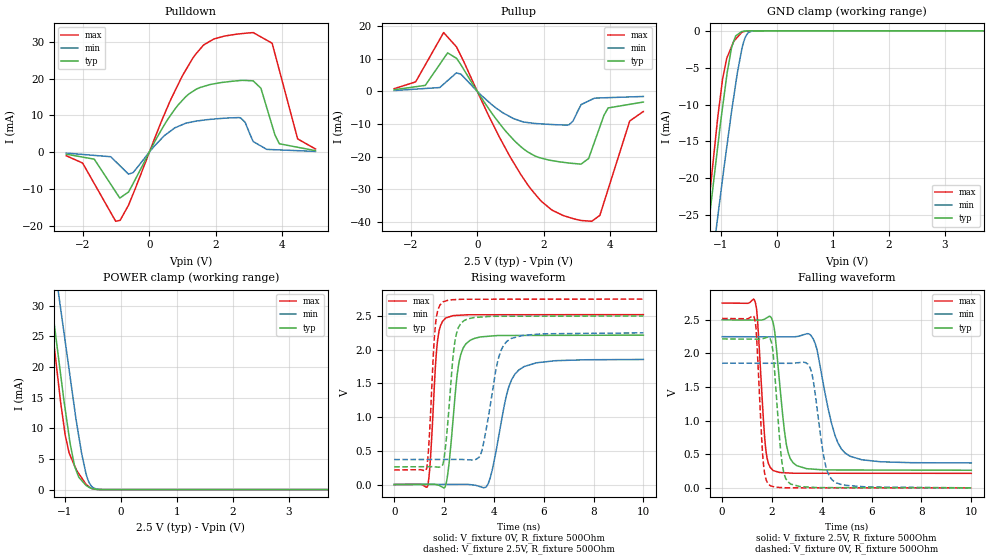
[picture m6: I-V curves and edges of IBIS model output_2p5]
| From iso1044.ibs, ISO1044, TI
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|   output_2p5 Model
[Model]   output_2p5
Model_type   3-state
Polarity   Inverting
Vmeas = 1.25
Vref = 0
Cref = 2pF
Rref = 100000
|   typ   min   max
C_comp   1.246pF   1.207pF   1.335pF
|C_comp_pullup   1.19pF   1.212pF   1.212pF
|C_comp_pulldown   1.131pF   1.152pF   1.158pF
|  Where Nom  PVT is Nominal Process, 2.5V,   27C
|   Fast PVT is Strong Process,  2.75,  -40C
|   Slow PVT is Weak Process,   2.25V,  150C
[Voltage Range]   2.5   2.25   2.75
|Junction Temperature
[Temperature Range]   27   150   -40
[Pullup Reference]   2.5   2.25   2.75
[Pulldown Reference]   -0   -0   0
[Power Clamp Reference]   2.5   2.25   2.75
[GND Clamp Reference]   0   0   0
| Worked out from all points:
|   slope of the pulldown table from 0 to 0.375 V, typ, clamps not added: 60.3 ohm
|   slope of the pullup table from 0 to 0.375 V, typ, clamps not added: 65.2 ohm
|   GND clamp passes 1 mA (typ) near -0.75 V on its own axis
|   POWER clamp passes 1 mA (typ) near -0.65 V on its own axis
|   falling waveform, V_fixture 2.5V, R_fixture 500Ohm: 20-80 % time 368ps typ, 664ps min, 250ps max; typ from 2.5 V to 0.262 V
|   rising waveform, V_fixture 0V, R_fixture 500Ohm: 20-80 % time 347ps typ, 615ps min, 233ps max; typ from 0 V to 2.22 V
|   rising waveform, V_fixture 2.5V, R_fixture 500Ohm: 20-80 % time 310ps typ, 531ps min, 212ps max; typ from 0.262 V to 2.5 V
|   falling waveform, V_fixture 0V, R_fixture 500Ohm: 20-80 % time 283ps typ, 428ps min, 209ps max; typ from 2.22 V to 0 V
[Pulldown]
|   Voltage   I(typ)   I(min)   I(max)
-2.5V     -577uA     -287.9uA   -1.006mA
-1.657V   -1.93mA    -903.9uA   -8.578mA
-879.3mV  -12.45mA   -3.763mA   -18.56mA
-486.8mV  -8.536mA   -5.561mA   -11.35mA
553.4mV   8.878mA    5.156mA    12.39mA
1.381V    16.92mA    8.373mA    26.47mA
2.746V    19.46mA    9.303mA    32.17mA
3.125V    19.37mA    2.86mA     32.5mA
3.696V    7.22mA     667.1uA    29.61mA
3.912V    2.258mA    586.3uA    22.27mA
4.464V    1.309mA    380.2uA    3.573mA
5V        388uA      180.2uA    845.5uA
[GND Clamp]
|   Voltage   I(typ)   I(min)   I(max)
-2.5V     -115.3mA   -116.6mA   -126.4mA
-1.497V   -45.2mA    -52.65mA   -45.36mA
-1.225V   -26.73mA   -35.65mA   -24.1mA
-1.057V   -15.78mA   -25.31mA   -11.83mA
-968.7mV  -10.36mA   -20.06mA   -6.529mA
-896.2mV  -6.193mA   -15.89mA   -3.763mA
-806.5mV  -2.199mA   -10.84mA   -2.1mA
-734.8mV  -686.4uA   -7.22mA    -1.127mA
-625mV    -98.47uA   -2.474mA   -201uA
-538.5mV  -20.04uA   -530.7uA   -38.58uA
-416.7mV  -957.2nA   -25.09uA   -1.059uA
5V        0A         0A         0A
[Pullup]
|   Voltage   I(typ)   I(min)   I(max)
-2.5V     504.9uA    255.7uA    828.2uA
-1.855V   1.423mA    688.6uA    2.91mA
-1.013V   10.01mA    2.217mA    18.02mA
-489.1mV  8.086mA    5.245mA    10.84mA
1.515V    -18.52mA   -9.543mA   -28.54mA
2.76V     -21.95mA   -10.26mA   -38.59mA
3.125V    -22.29mA   -4.049mA   -39.56mA
3.352V    -20.57mA   -2.944mA   -39.73mA
3.69V     -10.88mA   -2.009mA   -38mA
3.939V    -5.079mA   -1.924mA   -30mA
4.589V    -3.972mA   -1.703mA   -9.094mA
5V        -3.272mA   -1.563mA   -6.145mA
[POWER Clamp]
|   Voltage   I(typ)   I(min)   I(max)
-2.5V     128.9mA    131.9mA    138mA
-1.51V    51.07mA    59.94mA    50.15mA
-1.243V   30.77mA    41.03mA    27.33mA
-1.116V   21.48mA    31.98mA    17.2mA
-995.9mV  13.05mA    24.1mA     8.839mA
-926.6mV  8.645mA    19.55mA    5.963mA
-830.5mV  3.863mA    13.25mA    3.946mA
-703.7mV  1.504mA    5.938mA    1.939mA
-571.6mV  367.3uA    1.204mA    444.5uA
-470.7mV  96.86uA    197.6uA    59.09uA
-303.6mV  856.2nA    6.608uA    5.542uA
5V        0A         0A         0A
[Ramp]
R_load = 500
|   typ   min   max
dV/dt_r   1.32944/3.44254e-10   1.11276/6.08998e-10   1.51209/2.31266e-10
dV/dt_f   1.34275/3.66094e-10   1.12742/6.60572e-10   1.52035/2.48834e-10
[Falling Waveform]
V_fixture = 2.5V
V_fixture_min = 2.25V
V_fixture_max = 2.75V
R_fixture = 500Ohm
C_fixture = 0F
|   Time   V(typ)   V(min)   V(max)
0s        2.5V       2.25V      2.75V
1.327ns   2.497V     2.248V     2.768V
1.745ns   2.52V      2.248V     599.3mV
2.045ns   2.46V      2.247V     260.3mV
2.571ns   664.8mV    2.247V     223.3mV
2.981ns   333.5mV    2.251V     217.8mV
3.733ns   276.2mV    2.15V      217.6mV
4.389ns   266.3mV    962.5mV    217.4mV
4.929ns   265.9mV    520.9mV    217.3mV
10ns      262.1mV    370.6mV    216.1mV
[Rising Waveform]
V_fixture = 0V
V_fixture_min = 0V
V_fixture_max = 0V
R_fixture = 500Ohm
C_fixture = 0F
|   Time   V(typ)   V(min)   V(max)
0s        -149.7nV   307.1uV    -128.4nV
1.341ns   2.6mV      1.279mV    -24.13mV
1.725ns   -5.249mV   1.557mV    2.084V
2.065ns   -10.42mV   1.803mV    2.468V
2.591ns   1.792V     2.184mV    2.51V
3.041ns   2.137V     -1.144mV   2.518V
3.78ns    2.199V     19.03mV    2.518V
4.509ns   2.211V     1.329V     2.518V
4.999ns   2.211V     1.699V     2.519V
10ns      2.216V     1.855V     2.52V
[Rising Waveform]
V_fixture = 2.5V
V_fixture_min = 2.25V
V_fixture_max = 2.75V
R_fixture = 500Ohm
C_fixture = 0F
|   Time   V(typ)   V(min)   V(max)
0s        262.1mV    370.6mV    216.1mV
1.298ns   264.3mV    371.2mV    232.3mV
1.647ns   261.8mV    371.4mV    2.339V
1.945ns   293mV      371.5mV    2.706V
2.431ns   2.108V     371.7mV    2.743V
2.801ns   2.431V     370.2mV    2.748V
3.463ns   2.484V     439.7mV    2.749V
4.13ns    2.496V     1.789V     2.749V
4.519ns   2.496V     2.123V     2.749V
10ns      2.5V       2.25V      2.75V
[Falling Waveform]
|Gnd
V_fixture = 0V
V_fixture_min = 0V
V_fixture_max = 0V
R_fixture = 500Ohm
C_fixture = 0F
|   Time   V(typ)   V(min)   V(max)
0s        2.216V     1.855V     2.52V
1.298ns   2.213V     1.854V     2.524V
1.656ns   2.223V     1.854V     367.2mV
1.915ns   2.225V     1.854V     36.89mV
2.411ns   356.6mV    1.854V     4.107mV
2.741ns   59.66mV    1.853V     1.033mV
3.563ns   9.554mV    1.754V     916.1uV
4.14ns    3.562mV    353.6mV    834uV
4.559ns   3.308mV    79.22mV    774.3uV
10ns      -182.6nV   307uV      -121.4nV
